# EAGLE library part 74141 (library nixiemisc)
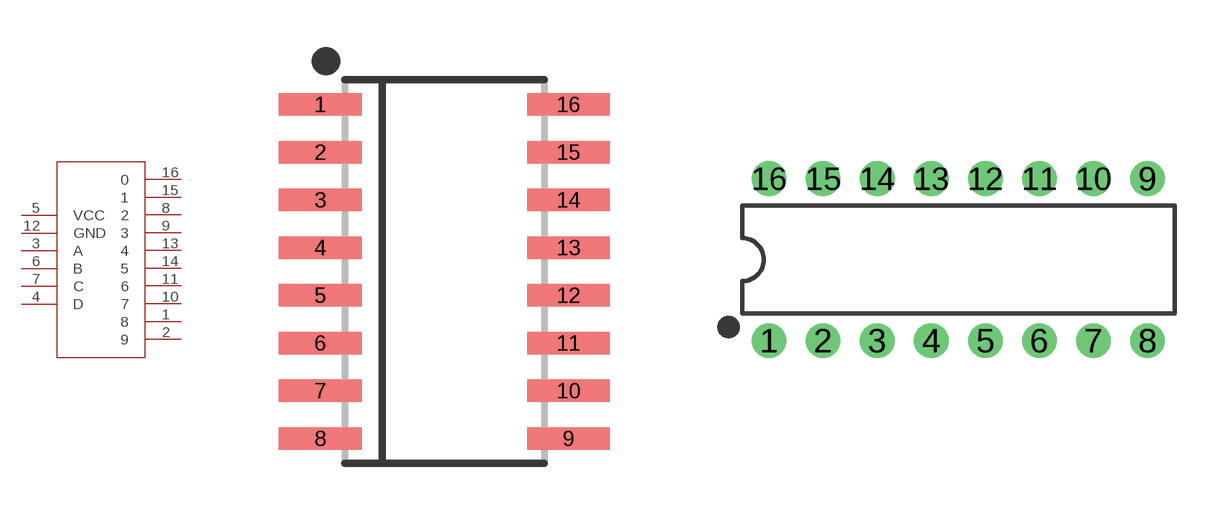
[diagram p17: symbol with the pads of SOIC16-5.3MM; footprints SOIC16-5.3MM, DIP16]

Designator prefix M

## 74141SOIC16  [SOIC16-5.3MM]
1  8  pas
2  9  pas
3  A  pas
4  D  pas
5  VCC  pwr
6  B  pas
7  C  pas
8  2  pas
9  3  pas
10  7  pas
11  6  pas
12  GND  pwr
13  4  pas
14  5  pas
15  1  pas
16  0  pas

## 74141DIP16  [DIP16]
Pads as for SOIC16-5.3MM

## Footprint SOIC16-5.3MM (pad centres in mm)
smd 2.2 x 0.6: 1 -3.3,4.445; 2 -3.3,3.175; 3 -3.3,1.905; 4 -3.3,0.635; 5 -3.3,-0.635; 6 -3.3,-1.905; 7 -3.3,-3.175; 8 -3.3,-4.445; 9 3.3,-4.445; 10 3.3,-3.175; 11 3.3,-1.905; 12 3.3,-0.635; 13 3.3,0.635; 14 3.3,1.905; 15 3.3,3.175; 16 3.3,4.445

## Footprint DIP16 (pad centres in mm)
Dual In Line Package
drill 0.813 pad 1.626: 1 -8.89,-3.81; 2 -6.35,-3.81; 3 -3.81,-3.81; 4 -1.27,-3.81; 5 1.27,-3.81; 6 3.81,-3.81; 7 6.35,-3.81; 8 8.89,-3.81; 9 8.89,3.81; 10 6.35,3.81; 11 3.81,3.81; 12 1.27,3.81; 13 -1.27,3.81; 14 -3.81,3.81; 15 -6.35,3.81; 16 -8.89,3.81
